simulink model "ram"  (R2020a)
settings: Solver=FixedStepDiscrete  StartTime=0.0  StopTime=Inf  FixedStep=0.01  RelTol=1e-3  EnableMultiTasking=on

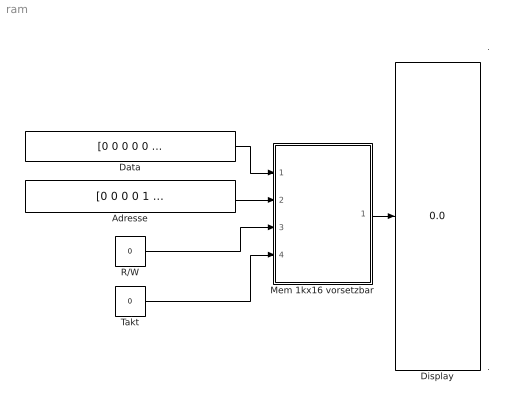
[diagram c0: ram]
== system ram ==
  note: .
  note: .
  Adresse : Constant  Value=[0 0 0 0 1 0 0 1 0 0]
  Data : Constant  Value=[0 0 0 0 0 0 1 0 0 0 1 0 0 1 1 1]
  Display : Display
  Mem 1kx16 vorsetzbar : Subsystem  mask(RAM){useFile=on}
      mask prompts: useFile "Inhalt von Datei lesen/schreiben"
      mask help: 1k x 16 Schreiblesespeicher liest optional von Datei ram.in (falls vorhanden) und schreibt nach ram.out
  R/W : Constant  Value=0
  Takt : Constant  Value=0
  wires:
  Data/1 -> Mem 1kx16 vorsetzbar/1(Data in)
  Adresse/1 -> Mem 1kx16 vorsetzbar/2(Address)
  R/W/1 -> Mem 1kx16 vorsetzbar/3(R/W)
  Takt/1 -> Mem 1kx16 vorsetzbar/4(" CLK")
  Mem 1kx16 vorsetzbar/1(Data out) -> Display/1

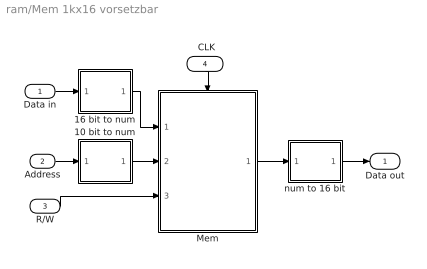
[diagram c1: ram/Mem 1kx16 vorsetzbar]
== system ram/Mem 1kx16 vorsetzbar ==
  note: .
  Data in : Inport  PortDimensions=16
  Address : Inport  Port=2  PortDimensions=10
  R/W : Inport  Port=3  PortDimensions=1
  " CLK" : Inport  Port=4  PortDimensions=1
  10 bit to num : Subsystem
  16 bit to num : Subsystem
  Mem : Subsystem  TreatAsAtomicUnit=on
  num to 16 bit : Subsystem
  Data out : Outport  InitialOutput=0
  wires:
  Data in/1 -> 16 bit to num/1(In)
  num to 16 bit/1(Out) -> Data out/1
  R/W/1 -> Mem/3(R/W)
  Address/1 -> 10 bit to num/1(In)
  " CLK"/1 -> Mem/Trigger
  16 bit to num/1(Out) -> Mem/1(Data in)
  10 bit to num/1(Out) -> Mem/2(Adress)
  Mem/1(Data out) -> num to 16 bit/1(In)

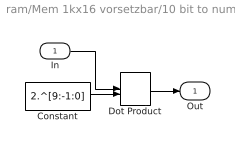
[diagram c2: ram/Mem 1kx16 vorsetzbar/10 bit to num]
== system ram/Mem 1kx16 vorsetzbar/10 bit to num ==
  In : Inport  PortDimensions=10
  Constant : Constant  Value=2.^[9:-1:0]
  Dot Product : DotProduct
  Out : Outport  InitialOutput=0
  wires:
  In/1 -> Dot Product/1
  Constant/1 -> Dot Product/2
  Dot Product/1 -> Out/1

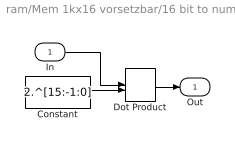
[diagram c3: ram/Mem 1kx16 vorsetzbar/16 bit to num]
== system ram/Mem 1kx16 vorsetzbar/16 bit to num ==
  note: .
  In : Inport  PortDimensions=16
  Constant : Constant  Value=2.^[15:-1:0]
  Dot Product : DotProduct
  Out : Outport  InitialOutput=0
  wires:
  Dot Product/1 -> Out/1
  Constant/1 -> Dot Product/2
  In/1 -> Dot Product/1

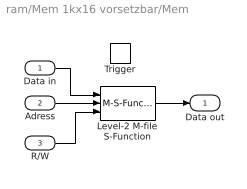
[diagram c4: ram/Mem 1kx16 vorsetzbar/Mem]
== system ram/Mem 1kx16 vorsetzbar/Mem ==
  note: .
  Data in : Inport  PortDimensions=1
  Adress : Inport  Port=2  PortDimensions=1
  R/W : Inport  Port=3  PortDimensions=1
  Trigger : TriggerPort  TriggerType=falling  VariantControl=Variant
  Level-2 M-file S-Function : M-S-Function  FunctionName=sfun_ram  Parameters=useFile
  Data out : Outport  InitialOutput=0
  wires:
  Adress/1 -> Level-2 M-file S-Function/2
  Data in/1 -> Level-2 M-file S-Function/1
  R/W/1 -> Level-2 M-file S-Function/3
  Level-2 M-file S-Function/1 -> Data out/1

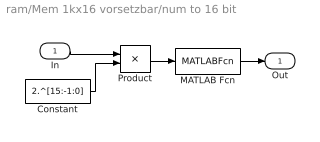
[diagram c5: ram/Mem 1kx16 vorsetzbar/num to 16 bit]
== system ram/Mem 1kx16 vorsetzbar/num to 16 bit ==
  note: .
  In : Inport  PortDimensions=1
  Constant : Constant  Value=2.^[15:-1:0]
  MATLAB Fcn : MATLABFcn  MATLABFcn=rem(floor(u),2)
  Product : Product  Inputs=*/  SaturateOnIntegerOverflow=on
  Out : Outport  InitialOutput=0
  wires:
  In/1 -> Product/1
  Constant/1 -> Product/2
  Product/1 -> MATLAB Fcn/1
  MATLAB Fcn/1 -> Out/1
